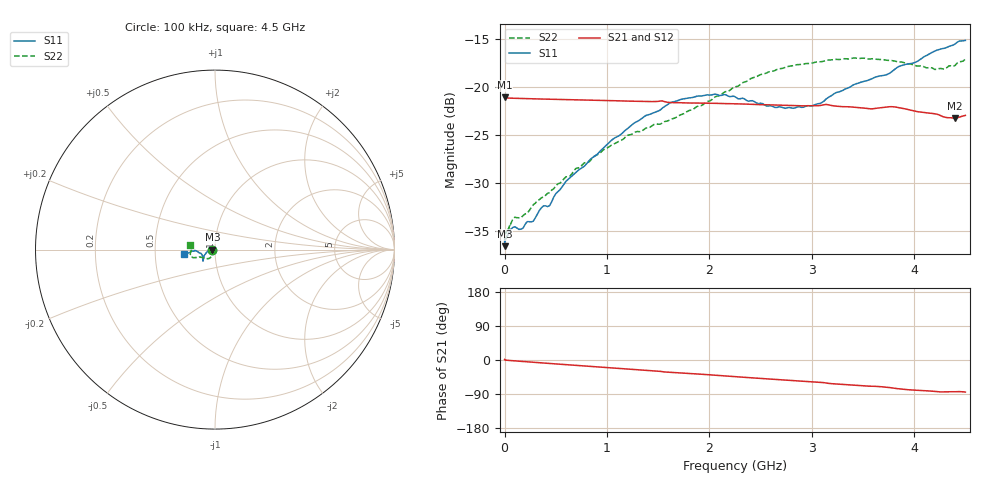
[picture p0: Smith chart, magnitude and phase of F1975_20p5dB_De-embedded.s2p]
! Integrated Device Technology
! Corporate Headquarters
! 6024 Silver Creek Valley Road
! San Jose, CA 95138  USA
! Phone:  1-408-284-8200
! Toll Free:  1-800-223-1366
! Webpage:  http://www.idt.com/
! Timing and RF Division
! 515 Groton Road, Suite 102
! Westford, MA 01886-6024
! Device:  F1975
! Description: 6-bit, 75 ohm, 0.5 dB Digital Step Attenuator
! Frequency:  5.0 MHz -  3.00 GHz
! Package:  4x4 mm QFN Plastic Package: 20 pin
! Ports:  2 RF, 11 DC
!  Pin  1  = D5 (16 dB)
!  Pin  2  = RF1  =  Port 1
!  Pin  3  = Serial Data In (DATA)
!  Pin  4  = Serial Clock (CLK)
!  Pin  5  = Serial Latch Enable (LE)
!  Pin  6  = VDD
!  Pin  7  = NC
!  Pin  8  = NC
!  Pin  9  = NC
!  Pin 10  = GND
!  Pin 11  = GND
!  Pin 12  = NC
!  Pin 13  = VMODE
!  Pin 14  = RF2  =  Port 2
!  Pin 15  = D4 (8 dB)
!  Pin 16  = D3 (4 dB)
!  Pin 17  = D2 (2 dB)
!  Pin 18  = NC
!  Pin 19  = D1 (1 dB)
!  Pin 20  = D0 (0.5 dB)
! State:  41
! Atten State:  20.5 dB
! Voltage:  +3.30 Volts
! Current:  0.564 mA
! Data:  The device was measured on a F1975 evaluation board which has
!  individual transmission lines to the RF pins.  Data was collected
!  using a calibrated network analyzer.  The evaluation board was
!  de-embedded using Automatic Fixture Removal (AFR).
!  The reference plane is the edge of the package pin.
! Misc:
!  Action Tracker AT0415
! Date Measured:  2018-02-08
! Date:  2018-03-26  MJV
! Note:
!  Integrated Device Technology supplies this data as a sample of measured
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# GHz S dB R 75
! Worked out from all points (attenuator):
!   291 points, 100 kHz to 4.5 GHz, reference 75 ohm
!   highest |S21| = -21.08 dB at 100 kHz (marker M1); lowest = -23.3 dB at 4.4 GHz (marker M2)
!   lowest |S11| = -36.6 dB at 100 kHz (marker M3), VSWR 1.03, Z = 72.8 - j0.0024 ohm
!   |S11| at or under -10 dB: start of sweep to end of sweep
!   |S22| runs from -36.2 to -17.0 dB; largest |S21 - S12| = 0.00016
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0.0001  -36.56 -179.9  -21.08 1.3  -21.08 1.2  -36.17 -178.5
0.008  -35.92 -178.4  -21.15 -0.1  -21.14 -0.0  -35.24 -175.5
0.08  -34.62 -176.0  -21.18 -1.9  -21.18 -1.9  -33.76 -164.2
0.16  -34.79 -176.7  -21.21 -3.5  -21.21 -3.6  -33.60 -151.0
0.22  -34.02 -178.9  -21.23 -4.8  -21.22 -4.8  -33.16 -144.6
0.28  -33.97 -179.8  -21.24 -6.0  -21.24 -6.0  -32.26 -141.0
0.36  -32.57 -179.8  -21.27 -7.6  -21.27 -7.6  -31.53 -133.1
0.44  -32.34 -178.9  -21.28 -9.1  -21.28 -9.1  -31.00 -127.4
0.6  -29.81 -175.2  -21.33 -12.3  -21.32 -12.3  -29.36 -123.1
0.76  -28.39 -168.2  -21.36 -15.4  -21.36 -15.4  -28.08 -120.9
1.26  -23.81 -152.9  -21.50 -25.1  -21.49 -25.1  -24.82 -121.7
1.52  -22.41 -144.2  -21.47 -30.0  -21.47 -30.0  -23.88 -128.8
1.62  -21.64 -142.6  -21.63 -32.3  -21.63 -32.3  -23.40 -132.1
1.88  -20.97 -138.7  -21.69 -36.8  -21.68 -36.8  -22.04 -143.8
2.26  -21.10 -138.0  -21.76 -44.0  -21.76 -44.0  -19.98 -155.0
2.64  -22.14 -147.3  -21.88 -51.2  -21.88 -51.2  -18.30 -158.6
3.02  -21.91 -164.0  -21.96 -58.0  -21.96 -58.0  -17.48 -161.4
3.42  -19.73 -175.3  -22.13 -66.8  -22.12 -66.8  -17.00 -167.3
3.76  -18.58 -175.8  -22.07 -72.8  -22.06 -72.8  -17.27 -174.0
4.2  -16.29 -172.8  -22.80 -82.8  -22.80 -82.8  -18.18 174.0
4.4  -15.54 -170.8  -23.25 -83.7  -23.24 -83.7  -17.77 170.7
4.5  -15.18 -172.6  -22.97 -84.7  -22.97 -84.7  -17.11 169.3
